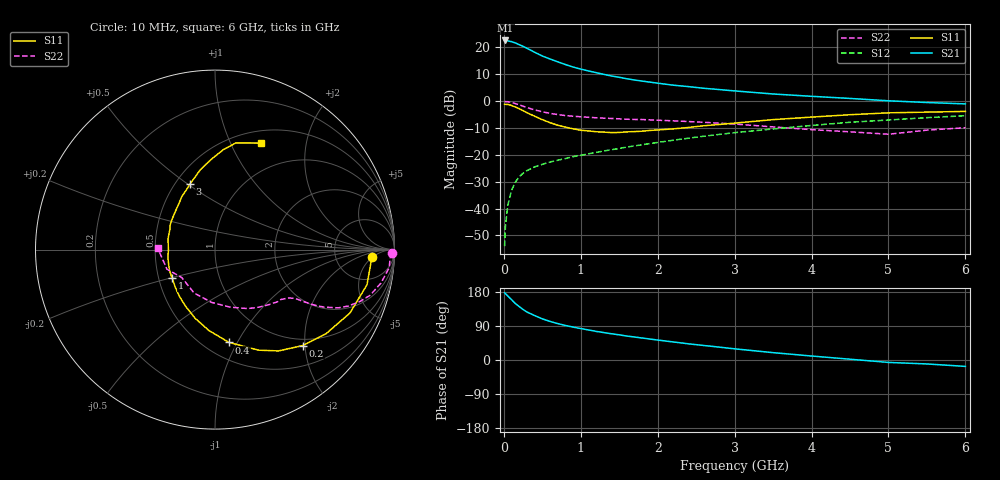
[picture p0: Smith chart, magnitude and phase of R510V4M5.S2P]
! SIEMENS Small Signal Semiconductors
! BFR183
! Si NPN RF Bipolar Junction Transistor in SOT23
! VCE = 10 V  IC = 4.5 mA
! Common Emitter S-Parameters:  May  1996
# GHz  S  MA  R  50
!  f  S11  S21  S12  S22
! GHz  MAG  ANG  MAG  ANG  MAG  ANG  MAG  ANG
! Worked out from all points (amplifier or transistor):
!   36 points, 10 MHz to 6 GHz, reference 50 ohm
!   highest |S21| = 22.6 dB at 20 MHz (marker M1)
!   |S21| within 3 dB of that: start of sweep to 306.1 MHz
!   unconditionally stable (mu >= 1): 1.165 GHz to 2.793 GHz
!   at 250 MHz: K = 0.38, MSG = 23.6 dB, |S12| = -26.8 dB
!   at 1.4 GHz: K = 1.05, MAG = 12.4 dB, |S12| = -18.1 dB
!   at 6 GHz: K = 0.87, MSG = 2.2 dB, |S12| = -5.4 dB
!   S11 on the Smith chart (normalised r, x): 10 MHz: 13, -5; 200 MHz: 0.87, -1.96; 400 MHz: 0.65, -0.93; 1 GHz: 0.59, -0.20; 3 GHz: 0.59, +0.51; 6 GHz: 0.65, +1.31
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0.01  0.8743 -2.6  13.36 177.7  0.002 82.2  0.9862 -1.1
0.02  0.8711 -5.3  13.47 175.2  0.0045 82.9  0.9781 -2.3
0.05  0.8692 -13.0  13.23 169.3  0.0113 83.5  0.9754 -6.0
0.1  0.8308 -25.2  12.79 159.3  0.0219 76.3  0.9434 -11.4
0.15  0.7763 -37.1  12.11 149.0  0.0311 70.7  0.9011 -16.4
0.2  0.7249 -47.5  11.25 141.0  0.0391 66.5  0.8552 -19.9
0.25  0.6664 -57.9  10.45 133.3  0.0455 62.8  0.8055 -23.0
0.3  0.611 -66.5  9.635 126.7  0.0508 60.3  0.7596 -25.3
0.4  0.5236 -81.3  8.125 117.3  0.0599 57.0  0.6873 -27.8
0.5  0.4522 -94.3  6.915 108.6  0.0667 55.3  0.6341 -29.2
0.6  0.3976 -106.3  6.091 101.8  0.0736 54.8  0.5924 -30.0
0.7  0.3561 -117.3  5.396 96.1  0.0794 54.9  0.5629 -30.6
0.8  0.3286 -126.8  4.799 91.1  0.0855 54.8  0.5389 -31.0
1  0.2872 -146.2  3.949 82.9  0.0981 55.7  0.5119 -31.9
1.1  0.2793 -155.2  3.652 79.3  0.1046 56.4  0.5006 -32.7
1.6  0.2681 167.1  2.611 63.2  0.1398 57.5  0.4609 -37.1
2.2  0.3046 137.2  1.984 47.7  0.1873 56.2  0.4303 -45.3
3  0.3898 111.1  1.55 29.5  0.2591 50.9  0.3748 -61.2
3.5  0.4532 100.3  1.359 19.4  0.3039 45.9  0.3319 -75.1
4.5  0.5589 85.2  1.123 2.1  0.4042 35.0  0.2685 -115.6
5.5  0.6247 72.2  0.943 -10.4  0.4932 22.9  0.2889 -157.8
6  0.6444 66.7  0.889 -16.9  0.5353 15.0  0.3202 178.3
